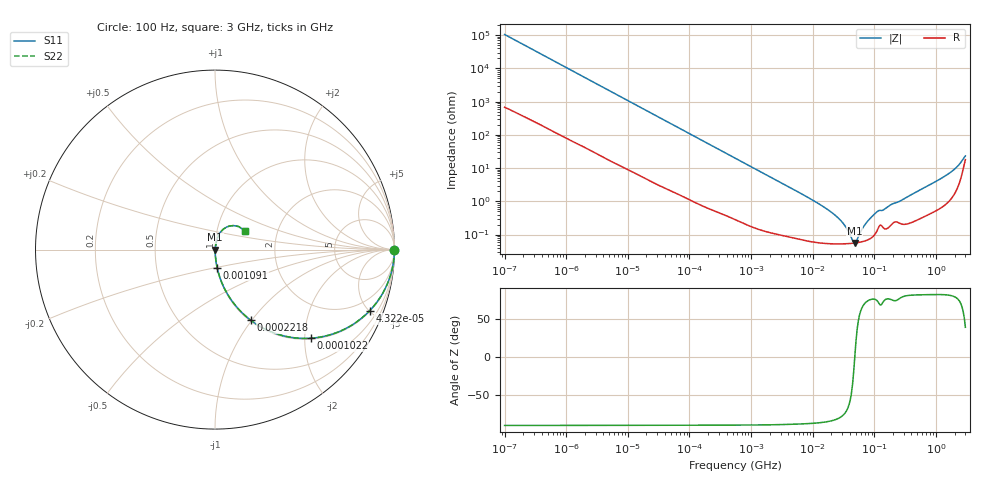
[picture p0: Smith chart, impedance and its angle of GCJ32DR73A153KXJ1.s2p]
!Murata Part Number: GCJ32DR73A153KXJ1
!These Parameters are Measured in Series Mode Connection
!Data Generated on Mar 13, 2026
!  o--ll--o
!Port1  Port2
!  o------o
!Operation Temp=25[degC], DC Bias Voltage=0[V]
!Freq. Start=100[Hz] Stop=3[GHz] 401[Steps]
# Hz S RI R 50
!Freq.(Hz) S11(Real) S11(Imag) S21(Real) S21(Imag) S12(Real) S12(Imag) S22(Real) S22(Imag)
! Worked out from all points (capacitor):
!   401 points, 100 Hz to 3 GHz, reference 50 ohm
!   read as one part in series: C = 15.1 nF near 109 Hz
!   lowest |Z| = 55.7 mohm at 48.15 MHz (marker M1)
!   series resonance near 48.06 MHz, so ESL is about 730 pH
!   S11 on the Smith chart (normalised r, x): 100 Hz: open; 43.22 kHz: 1.05, -5.03; 102.2 kHz: 1.02, -2.14; 221.8 kHz: 1.01, -0.99; 1.091 MHz: 1.00, -0.20; 3 GHz: 1.36, +0.30
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100  1 -0.000949  7e-06 0.000949  7e-06 0.000949  1 -0.000949
1788  0.9996 -0.0167  0.00041 0.0167  0.00041 0.0167  0.9996 -0.0167
9582  0.9914 -0.0881  0.00857 0.0881  0.00857 0.0881  0.9914 -0.0881
31977  0.918 -0.27  0.082 0.27  0.082 0.27  0.918 -0.27
43220  0.861 -0.3414  0.139 0.3414  0.139 0.3414  0.861 -0.3414
102221  0.5326 -0.4938  0.4674 0.4938  0.4674 0.4938  0.5326 -0.4938
221826  0.1992 -0.3937  0.8008 0.3937  0.8008 0.3937  0.1992 -0.3937
547723  0.0416 -0.1927  0.9584 0.1927  0.9584 0.1927  0.0416 -0.1927
1090550  0.0118 -0.1004  0.9882 0.1004  0.9882 0.1004  0.0118 -0.1004
9794414  0.000724 -0.0111  0.9993 0.0111  0.9993 0.0111  0.000724 -0.0111
2.635803e7  0.000532 -0.00302  0.9995 0.00302  0.9995 0.00302  0.000532 -0.00302
3.268714e7  0.000531 -0.00187  0.9995 0.00187  0.9995 0.00187  0.000531 -0.00187
4.418008e7  0.000547 -0.0004  0.9995 0.0004  0.9995 0.0004  0.000547 -0.0004
4.815176e7  0.000557 9.6e-06  0.9994 -9.6e-06  0.9994 -9.6e-06  0.000557 9.6e-06
5.248048e7  0.00057 0.000421  0.9994 -0.000421  0.9994 -0.000421  0.00057 0.000421
6.794454e7  0.000634 0.0017  0.9994 -0.0017  0.9994 -0.0017  0.000634 0.0017
8.79653e7  0.000788 0.00315  0.9992 -0.00315  0.9992 -0.00315  0.000788 0.00315
1.138854e8  0.00149 0.00486  0.9985 -0.00486  0.9985 -0.00486  0.00149 0.00486
1.751444e8  0.00176 0.00722  0.9982 -0.00722  0.9982 -0.00722  0.00176 0.00722
1.324213e9  0.00993 0.0527  0.9901 -0.0527  0.9901 -0.0527  0.00993 0.0527
2.219584e9  0.035 0.1025  0.965 -0.1025  0.965 -0.1025  0.035 0.1025
3e9  0.1654 0.1047  0.8346 -0.1047  0.8346 -0.1047  0.1654 0.1047
